INTERFACE I_Generator

METHOD M_Flash : BOOL
VAR_INPUT
END_VAR
END_METHOD

PROPERTY P_Cycletime : TIME
GET
END_GET
SET
END_SET
END_PROPERTY

PROPERTY P_Vendor : String
GET
END_GET
END_PROPERTY

END_INTERFACE
